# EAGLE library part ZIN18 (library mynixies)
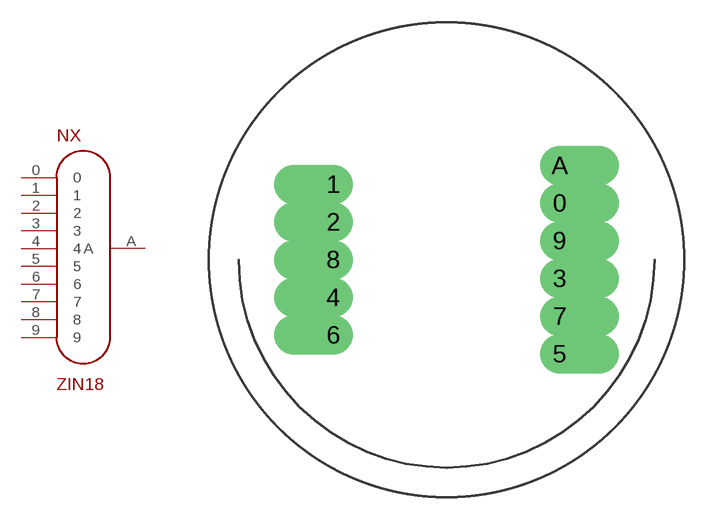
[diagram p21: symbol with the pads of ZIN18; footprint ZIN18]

Designator prefix NX

## ZIN18  [ZIN18]
0  0  pas
1  1  pas
2  2  pas
3  3  pas
4  4  pas
5  5  pas
6  6  pas
7  7  pas
8  8  pas
9  9  pas
A  A  pas

## Footprint ZIN18 (pad centres in mm)
drill 1.778 pad 1.956 offset: 0 7.62,3.81; 1 -7.62,5.08; 2 -7.62,2.54; 3 7.62,-1.27; 4 -7.62,-2.54; 5 7.62,-6.35; 6 -7.62,-5.08; 7 7.62,-3.81; 8 -7.62,0; 9 7.62,1.27; A 7.62,6.35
